| TEXAS INSTRUMENTS INCORPORATED
| Standard Linear and Logic Group
| IBIS Model of SN74CBTLV3384
| LOW-VOLTAGE 10-BIT FET BUS SWITCH
| This file contains package information for the following:
|  SSOP 24-pin (DBQ) package as [Component] CBTLV3384_DBQ
|  TVSOP 24-pin (DGV) package as [Component] CBTLV3384_DGV
|  SOIC 24-pin (DW) package as [Component] CBTLV3384_DW
|  TSSOP 24-pin (PW) package as [Component] CBTLV3384_PW
| This device can be powered at the following Vccs:
|  2.5 volt Vcc
|  3.3 volt Vcc
| This file provides unique models under the [Model Selector] for each Vcc.
| For operation at a specific Vcc, select the appropriate model after each
| [Model Selector] keyword.
[IBIS Ver]   3.2
[Comment char]  |_char
[File Name]   sn74cbtlv3384.ibs
[File Rev]   1.2 | a_die
[Date]   April 6, 2005
[Source]   Data created from TI-SPICE simulations at TI-SLL.
[Notes]   The following is an IBIS list for the CBTLV3384.
   Please contact sllibis@ti.com with questions and
   comments concerning SLL IBIS models.
   - FILE REV HISTORY
   - 1.1 Release IBIS
   - 1.2 Syntax corrections made. 04/06/05
   - Power clamp data deleted as there is no power-clamp diode.
   - Non-monotonic data due to FET characteristics.
[Disclaimer] Property of Texas Instruments Incorporated.  Unauthorized
   reproduction and/or distribution is strictly prohibited.
   This product is protected under copyright law.
   Created  2003, (C) Copyright  2003, Texas Instruments
   Incorporated, All Rights Reserved
   UNLESS THERE IS A SIGNED, WRITTEN AGREEMENT TO THE
   CONTRARY, TEXAS INSTRUMENTS (TI) IS PROVIDING THE IBIS
   MODELS  AND WITHOUT ANY WARRANTY, EXPRESSED OR
   IMPLIED.  TI assumes no liability for:
   1) the accuracy of the IBIS models provided to your
   company;
   2) the proper functioning of these IBIS Models in your
   design or for any resulting applications; or
   3) infringement of patents, copyrights or intellectual
   property rights resulting from your use of these IBIS
   models.
   TI provides IBIS Models as a service to our customers.
   You and your company shall not distribute, sell or give
   these models to anyone else without prior written
   permission from TI.
   TI reserves the right to make changes to our products or
   to discontinue any semiconductor product or service
   without notice, and advises our customers to obtain the
   latest version of relevant information to verify, before
   placing orders, that the information being relied on is
   current.
   Please be aware that your receipt and use of the IBIS
   information provided shall serve as acceptance of these
   terms and conditions.  If you do not accept these terms,
   you should return or destroy the IBIS models and any
   other accompanying information immediately.
| Component CBTLV3384_DBQ 24-pin SSOP
[Component]   CBTLV3384_DBQ
[Manufacturer]   Texas Instruments, Inc.
[Package]
|   typ   min   max
R_pkg   4.400e-02   3.100e-02   6.600e-02
L_pkg   3.074e-09   2.348e-09   4.044e-09
C_pkg   3.220e-13   2.340e-13   4.460e-13
[Pin]   signal_name   model_name   R_pin   L_pin   C_pin
1   N1OE   CBTLV3384_NOE   6.500e-02   4.044e-09   4.290e-13
2   1B1   CBTLV3384_IO   6.600e-02   3.824e-09   4.460e-13
3   1A1   CBTLV3384_IO   3.100e-02   3.011e-09   3.210e-13
4   1A2   CBTLV3384_IO   3.200e-02   2.699e-09   2.590e-13
5   1B2   CBTLV3384_IO   3.500e-02   2.519e-09   2.450e-13
6   1B3   CBTLV3384_IO   3.500e-02   2.348e-09   2.340e-13
7   1A3   CBTLV3384_IO   3.500e-02   2.348e-09   2.340e-13
8   1A4   CBTLV3384_IO   3.500e-02   2.518e-09   2.450e-13
9   1B4   CBTLV3384_IO   3.200e-02   2.699e-09   2.590e-13
10   1B5   CBTLV3384_IO   3.100e-02   3.011e-09   3.210e-13
11   1A5   CBTLV3384_IO   6.600e-02   3.824e-09   4.460e-13
12   GND   GND   6.500e-02   4.044e-09   4.290e-13
13   N2OE   CBTLV3384_NOE   6.500e-02   4.044e-09   4.290e-13
14   2A1   CBTLV3384_IO   6.600e-02   3.824e-09   4.460e-13
15   2B1   CBTLV3384_IO   3.100e-02   3.011e-09   3.210e-13
16   2B2   CBTLV3384_IO   3.200e-02   2.699e-09   2.590e-13
17   2A2   CBTLV3384_IO   3.500e-02   2.518e-09   2.450e-13
18   2A3   CBTLV3384_IO   3.500e-02   2.348e-09   2.340e-13
19   2B3   CBTLV3384_IO   3.500e-02   2.348e-09   2.340e-13
20   2B4   CBTLV3384_IO   3.500e-02   2.518e-09   2.450e-13
21   2A4   CBTLV3384_IO   3.200e-02   2.699e-09   2.590e-13
22   2A5   CBTLV3384_IO   3.100e-02   3.011e-09   3.210e-13
23   2B5   CBTLV3384_IO   6.600e-02   3.824e-09   4.460e-13
24   VCC   POWER   6.500e-02   4.044e-09   4.290e-13
| Component CBTLV3384_DGV 24-pin TVSOP
[Component]   CBTLV3384_DGV
[Manufacturer]   Texas Instruments, Inc.
[Package]
|   typ   min   max
R_pkg   4.300e-02   3.900e-02   4.700e-02
L_pkg   2.601e-09   2.312e-09   3.626e-09
C_pkg   3.580e-13   2.770e-13   5.950e-13
[Pin]   signal_name   model_name   R_pin   L_pin   C_pin
1   N1OE   CBTLV3384_NOE   4.300e-02   3.625e-09   5.950e-13
2   1B1   CBTLV3384_IO   4.000e-02   2.656e-09   4.020e-13
3   1A1   CBTLV3384_IO   3.900e-02   2.338e-09   3.080e-13
4   1A2   CBTLV3384_IO   4.600e-02   2.354e-09   2.770e-13
5   1B2   CBTLV3384_IO   4.500e-02   2.312e-09   2.850e-13
6   1B3   CBTLV3384_IO   4.700e-02   2.318e-09   2.820e-13
7   1A3   CBTLV3384_IO   4.700e-02   2.318e-09   2.820e-13
8   1A4   CBTLV3384_IO   4.500e-02   2.312e-09   2.850e-13
9   1B4   CBTLV3384_IO   4.600e-02   2.353e-09   2.780e-13
10   1B5   CBTLV3384_IO   3.900e-02   2.338e-09   3.080e-13
11   1A5   CBTLV3384_IO   4.100e-02   2.660e-09   4.020e-13
12   GND   GND   4.300e-02   3.625e-09   5.950e-13
13   N2OE   CBTLV3384_NOE   4.400e-02   3.626e-09   5.940e-13
14   2A1   CBTLV3384_IO   4.000e-02   2.658e-09   4.020e-13
15   2B1   CBTLV3384_IO   3.900e-02   2.343e-09   3.110e-13
16   2B2   CBTLV3384_IO   4.600e-02   2.353e-09   2.780e-13
17   2A2   CBTLV3384_IO   4.500e-02   2.312e-09   2.850e-13
18   2A3   CBTLV3384_IO   4.700e-02   2.319e-09   2.820e-13
19   2B3   CBTLV3384_IO   4.700e-02   2.319e-09   2.820e-13
20   2B4   CBTLV3384_IO   4.500e-02   2.312e-09   2.850e-13
21   2A4   CBTLV3384_IO   4.600e-02   2.353e-09   2.780e-13
22   2A5   CBTLV3384_IO   3.900e-02   2.337e-09   3.080e-13
23   2B5   CBTLV3384_IO   4.000e-02   2.658e-09   4.020e-13
24   VCC   POWER   4.400e-02   3.626e-09   5.950e-13
| Component CBTLV3384_DW 24-pin SOIC
[Component]   CBTLV3384_DW
[Manufacturer]   Texas Instruments, Inc.
[Package]
|   typ   min   max
R_pkg   3.700e-02   3.000e-02   4.700e-02
L_pkg   5.146e-09   3.993e-09   6.885e-09
C_pkg   7.580e-13   5.120e-13   1.067e-12
[Pin]   signal_name   model_name   R_pin   L_pin   C_pin
1   N1OE   CBTLV3384_NOE   3.900e-02   6.885e-09   1.067e-12
2   1B1   CBTLV3384_IO   4.200e-02   5.950e-09   9.580e-13
3   1A1   CBTLV3384_IO   4.700e-02   5.317e-09   7.910e-13
4   1A2   CBTLV3384_IO   3.100e-02   4.651e-09   6.110e-13
5   1B2   CBTLV3384_IO   3.000e-02   3.993e-09   5.120e-13
6   1B3   CBTLV3384_IO   3.000e-02   4.083e-09   6.110e-13
7   1A3   CBTLV3384_IO   3.000e-02   4.083e-09   6.110e-13
8   1A4   CBTLV3384_IO   3.000e-02   3.993e-09   5.120e-13
9   1B4   CBTLV3384_IO   3.100e-02   4.652e-09   6.110e-13
10   1B5   CBTLV3384_IO   4.700e-02   5.317e-09   7.910e-13
11   1A5   CBTLV3384_IO   4.200e-02   5.950e-09   9.590e-13
12   GND   GND   3.900e-02   6.885e-09   1.067e-12
13   N2OE   CBTLV3384_NOE   3.900e-02   6.885e-09   1.067e-12
14   2A1   CBTLV3384_IO   4.200e-02   5.950e-09   9.590e-13
15   2B1   CBTLV3384_IO   4.700e-02   5.317e-09   7.910e-13
16   2B2   CBTLV3384_IO   3.100e-02   4.652e-09   6.110e-13
17   2A2   CBTLV3384_IO   3.000e-02   3.993e-09   5.120e-13
18   2A3   CBTLV3384_IO   3.000e-02   4.083e-09   6.100e-13
19   2B3   CBTLV3384_IO   3.000e-02   4.083e-09   6.100e-13
20   2B4   CBTLV3384_IO   3.000e-02   3.993e-09   5.120e-13
21   2A4   CBTLV3384_IO   3.100e-02   4.651e-09   6.110e-13
22   2A5   CBTLV3384_IO   4.700e-02   5.317e-09   7.910e-13
23   2B5   CBTLV3384_IO   4.200e-02   5.950e-09   9.580e-13
24   VCC   POWER   3.900e-02   6.885e-09   1.067e-12
| Component CBTLV3384_PW 24-pin TSSOP
[Component]   CBTLV3384_PW
[Manufacturer]   Texas Instruments, Inc.
[Package]
|   typ   min   max
R_pkg   3.900e-02   3.000e-02   4.600e-02
L_pkg   2.685e-09   2.367e-09   3.177e-09
C_pkg   3.200e-13   2.520e-13   4.340e-13
[Pin]   signal_name   model_name   R_pin   L_pin   C_pin
1   N1OE   CBTLV3384_NOE   3.700e-02   3.153e-09   4.340e-13
2   1B1   CBTLV3384_IO   3.400e-02   2.629e-09   3.410e-13
3   1A1   CBTLV3384_IO   3.200e-02   2.860e-09   3.470e-13
4   1A2   CBTLV3384_IO   4.200e-02   2.741e-09   2.900e-13
5   1B2   CBTLV3384_IO   4.600e-02   2.600e-09   2.620e-13
6   1B3   CBTLV3384_IO   4.300e-02   2.414e-09   2.660e-13
7   1A3   CBTLV3384_IO   4.200e-02   2.367e-09   2.620e-13
8   1A4   CBTLV3384_IO   4.400e-02   2.461e-09   2.520e-13
9   1B4   CBTLV3384_IO   4.200e-02   2.543e-09   2.740e-13
10   1B5   CBTLV3384_IO   3.000e-02   2.616e-09   3.320e-13
11   1A5   CBTLV3384_IO   3.700e-02   2.670e-09   3.460e-13
12   GND   GND   3.900e-02   3.177e-09   4.330e-13
13   N2OE   CBTLV3384_NOE   3.700e-02   3.111e-09   4.310e-13
14   2A1   CBTLV3384_IO   3.700e-02   2.656e-09   3.450e-13
15   2B1   CBTLV3384_IO   3.100e-02   2.739e-09   3.400e-13
16   2B2   CBTLV3384_IO   4.200e-02   2.649e-09   2.820e-13
17   2A2   CBTLV3384_IO   4.600e-02   2.532e-09   2.570e-13
18   2A3   CBTLV3384_IO   4.400e-02   2.425e-09   2.660e-13
19   2B3   CBTLV3384_IO   4.400e-02   2.425e-09   2.660e-13
20   2B4   CBTLV3384_IO   4.600e-02   2.532e-09   2.570e-13
21   2A4   CBTLV3384_IO   4.200e-02   2.648e-09   2.820e-13
22   2A5   CBTLV3384_IO   3.100e-02   2.738e-09   3.390e-13
23   2B5   CBTLV3384_IO   3.600e-02   2.653e-09   3.440e-13
24   VCC   POWER   3.700e-02   3.110e-09   4.310e-13
[Series Switch Groups]
| Function Group States
On  1 /   | 1A1-1A5->1B1-1B5 NOE1 LOW
On  2 /   | 2A1-2A5->2B1-2B5 NOE2 LOW
On  1 2 /   | Enable Both
[Series Pin Mapping]   pin_2   model_name   function_table_group
3   2   CBTLV3384_IO_25_S   1
| 3   2   CBTLV3384_IO_33_S   1
4   5   CBTLV3384_IO_25_S   1
| 4   5   CBTLV3384_IO_33_S   1
7   6   CBTLV3384_IO_25_S   1
| 7   6   CBTLV3384_IO_33_S   1
8   9   CBTLV3384_IO_25_S   1
| 8   9   CBTLV3384_IO_33_S   1
11   10   CBTLV3384_IO_25_S   1
| 11   10   CBTLV3384_IO_33_S   1
14   15   CBTLV3384_IO_25_S   2
| 14   15   CBTLV3384_IO_33_S   2
17   16   CBTLV3384_IO_25_S   2
| 17   16   CBTLV3384_IO_33_S   2
18   19   CBTLV3384_IO_25_S   2
| 18   19   CBTLV3384_IO_33_S   2
21   20   CBTLV3384_IO_25_S   2
| 21   20   CBTLV3384_IO_33_S   2
22   23   CBTLV3384_IO_25_S   2
| 22   23   CBTLV3384_IO_33_S   2
| Model CBTLV3384_NOE
[Model Selector]   CBTLV3384_NOE
CBTLV3384_NOE_25   2.5 volt Vcc
CBTLV3384_NOE_33   3.3 volt Vcc
| Model CBTLV3384_IO
[Model Selector]   CBTLV3384_IO
CBTLV3384_IO_25   2.5 volt Vcc
CBTLV3384_IO_33   3.3 volt Vcc
| Model CBTLV3384_IO_S
[Model Selector]   CBTLV3384_IO_S
CBTLV3384_IO_33_S   3.3 volt Vcc_S
CBTLV3384_IO_25_S   2.5 volt Vcc_S
[Model]   CBTLV3384_IO_25_S
Model_type  Series_switch
| variable   typ   min   max
C_comp   0   0   0
[Temperature Range]   40   100   -40
| Ambient temperature   25   85   -40
[Voltage range]   2.5   2.3   2.7
[On]
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[Off]
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[Model]   CBTLV3384_IO_33_S
Model_type  Series_switch
| variable   typ   min   max
C_comp   0   0   0
[Temperature Range]   40   100   -40
| Ambient temperature   25   85   -40
[Voltage range]   3.3   3   3.6
[On]
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[Off]
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| Models and submodels in the file (6): CBTLV3384_NOE_25 (Input), CBTLV3384_NOE_33 (Input), CBTLV3384_IO_25_S (Series_switch), CBTLV3384_IO_25 (Terminator), CBTLV3384_IO_33_S (Series_switch), CBTLV3384_IO_33 (Terminator)
